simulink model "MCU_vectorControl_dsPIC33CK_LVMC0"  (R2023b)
settings: Solver=FixedStepDiscrete  StartTime=0.0  StopTime=10.0  FixedStep=5e-5  RelTol=1e-3  EnableMultiTasking=on
undefined symbols (not defined in the file or in its folder): A0, A4, ADC, address, also, AN0, AN1, as, B0, B2, below, Bias1, Bias2, bit, bits, BOR, C12, C13, C14, C7, C8, cause, Code, Communicate, control, counter, Custom, D11, D12, D13, D14, D2, D5, D6, D7, D9, dead, default, deviced, diff, disasserted, DiscIntNeverNeededParam, ECIO, ensure, events, faster, HS3, I, I2C, I2C1, I2C2, I2C3, illegalInstruction, Interval, inverter, is, IsSigned1, IsSigned2, kHz, Lowest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
libraries: simulink x55, MCHP_Blockset x25
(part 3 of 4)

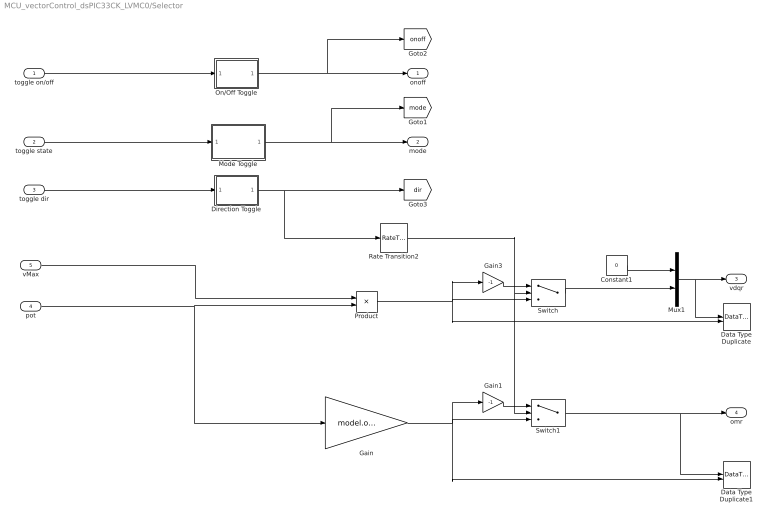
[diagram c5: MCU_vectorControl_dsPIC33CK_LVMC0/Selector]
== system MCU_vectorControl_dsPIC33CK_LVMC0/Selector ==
  toggle on/off : Inport  SampleTime=.01
  toggle state : Inport  Port=2  SampleTime=.01
  toggle dir : Inport  Port=3  SampleTime=.01
  pot : Inport  Port=4
  vMax : Inport  Port=5
  Constant1 : Constant  Value=0  OutDataTypeStr=Inherit: Inherit via back propagation
  Data Type Duplicate : DataTypeDuplicate
  Data Type Duplicate1 : DataTypeDuplicate
  Direction Toggle : Subsystem
  Gain : Gain  Gain=model.omegaMax  OutDataTypeStr=Inherit: Inherit via back propagation
  Gain1 : Gain  Gain=-1  OutDataTypeStr=Inherit: Inherit via back propagation  SaturateOnIntegerOverflow=on
  Gain3 : Gain  Gain=-1  OutDataTypeStr=Inherit: Inherit via back propagation  SaturateOnIntegerOverflow=on
  Mode Toggle : Subsystem
  Mux1 : Mux  Inputs=2
  On/Off Toggle : Subsystem
  Product : Product
  Rate Transition2 : RateTransition  Integrity=off  OutPortSampleTime=0.001
  Switch : Switch  Criteria=u2 > Threshold  OutDataTypeStr=Inherit: Inherit via back propagation
  Switch1 : Switch  Criteria=u2 > Threshold  OutDataTypeStr=Inherit: Inherit via back propagation
  onoff : Outport
  mode : Outport  Port=2
  vdqr : Outport  Port=3  VectorParamsAs1DForOutWhenUnconnected=off
  omr : Outport  Port=4  VectorParamsAs1DForOutWhenUnconnected=off
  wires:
  Switch1/1 -> omr/1, Data Type Duplicate1/1
  Direction Toggle/1(Toggle) -> Rate Transition2/1, [dir]
  Gain1/1 -> Switch1/1
  Gain/1 -> Gain1/1, Switch1/3, Data Type Duplicate1/2
  Product/1 -> Data Type Duplicate/2, Switch/3, Gain3/1
  Mux1/1 -> Data Type Duplicate/1, vdqr/1
  Constant1/1 -> Mux1/1
  toggle on/off/1 -> On/Off Toggle/1(in)
  On/Off Toggle/1(Toggle) -> [onoff], onoff/1
  Mode Toggle/1(Mode) -> [mode], mode/1
  toggle state/1 -> Mode Toggle/1(state)
  toggle dir/1 -> Direction Toggle/1(in)
  Gain3/1 -> Switch/1
  Switch/1 -> Mux1/2
  vMax/1 -> Product/1
  Rate Transition2/1 -> Switch/2, Switch1/2
  pot/1 -> Gain/1, Product/2

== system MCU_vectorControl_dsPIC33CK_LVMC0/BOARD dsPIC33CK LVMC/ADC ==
  ADC dsPIC High Speed SAR Motor Currents : MCHP_Blockset/Analog IO/ADC dsPIC High Speed SAR  ACLKCON=Optimized for PWM resolution & ADC conversion speed  ADC_FRACT=Fractional (left aligned)  ADC_NRE=off  DMA_Size=Single trigger - (default)  ADC_Synchronisation=Triggered by custom source  ADC_Trig_TXT=PWM1 Trigger 1  ADC_TrigTimeStep=Trig model step after all sample from this block are converted  ADC_TrigInfo=0  SampleTime=50e-6  S_INPUT=[]  S_INPUT_Size=[]  S_OUTPUT="[5  5]"  S_OUTPUT_Size="[1  1]"  S_ListCustomDatatype=S.S_ListCustomDatatype={};  MCHP_USER_INTERRUPTS={ADCAN0}{ADCBUF0}{ADC Data 0 Ready}{VectorName(ADCAN0Interrupt) Priority(-1) RegisterReadClear(ADCBUF0)Config_BitSet(ADIELbits.IE0) };{ADCAN1}{ADCBUF1}{ADC Data 1 Ready}{VectorName(ADCAN1Interrupt) Priority(-1) RegisterReadClear(ADCBUF1)Config_BitSet(ADIELbits.IE1) };  MCHP_PORT={Analog Input 0}{AN0}15:2:A0;{Analog Input 1}{AN1}15:2:B2;  MCHP_MASTERLINK=MCU_vectorControl_dsPIC33CK_LVMC0/BOARD dsPIC33CK LVMC/Microchip Master  MCHP_CRC=4309706  ADC_Info=Total Time = 640(ns)  ADC0_pin_TXT=AN0 / A0 / Pin[16]  ADC0_R="< 5    kOhm"  ADC0_res=12 bits  ADC0_signed=signed 16 bits  ADC0_FILTER=No Oversampling  ADC0_FILTER_nSamples=256 samples  ADC0_STRGEN=Start sampling followed by conversion  ADC0_STRGEN_on=Start sampling followed by conversion  ADC0_SSAMPEN=off  ADC0_Info=tSmp_min=260(ns) x 1 = 260(ns) ; tConv=370(ns) x 1 = 370(ns) ; TOTAL=640(ns)  ADC1_pin_TXT=AN1 / B2 / Pin[41]  ADC1_R="< 5    kOhm"  ADC1_res=12 bits  ADC1_signed=signed 16 bits  ADC1_FILTER=No Oversampling  ADC1_FILTER_nSamples=128 samples  ADC1_STRGEN=Start sampling followed by conversion  ADC1_STRGEN_on=Start sampling followed by conversion  ADC1_SSAMPEN=off  ADC1_Info=tSmp_min=260(ns) x 1 = 260(ns) ; tConv=370(ns) x 1 = 370(ns) ; TOTAL=640(ns)  ADC2_pin_TXT=Not used  ADC2_R="< 5    kOhm"  ADC2_res=12 bits  ADC2_signed=signed 16 bits  ADC2_FILTER=No Oversampling  ADC2_FILTER_nSamples=256 samples  ADC2_STRGEN=End sampling and start conversion  ADC2_STRGEN_on=Start sampling followed by conversion  ADC2_SSAMPEN=on  ADC2_Info=tSmp_min=14.706(ns) x 0 = 0(s) ; tConv=154.41(ns) x 0 = 0(s) ; TOTAL=0(s)  ADC3_pin_TXT=Not used  ADC3_R="< 10   kOhm"  ADC3_res=12 bits  ADC3_signed=signed 16 bits  ADC3_FILTER=Burst convert of n samples are Summed  ADC3_FILTER_nSamples=64 samples  ADC3_STRGEN=End sampling and start conversion  ADC3_STRGEN_on=Start sampling followed by conversion  ADC3_SSAMPEN=on  ADC3_Info=tSmp_min=14.706(ns) x 0 = 0(s) ; tConv=154.41(ns) x 0 = 0(s) ; TOTAL=0(s)  ADC4_pin_TXT=Not used  ADC4_R=< 200 Ohm  ADC4_res=12 bits  ADC4_signed=unsigned 16 bits  ADC4_FILTER=No Oversampling  ADC4_FILTER_nSamples=256 samples  ADC4_STRGEN=End sampling and start conversion  ADC4_STRGEN_on=Start sampling followed by conversion  ADC4_SSAMPEN=off  ADC4_Info=tSmp_min=14.706(ns) x 0 = 0(s) ; tConv=154.41(ns) x 0 = 0(s) ; TOTAL=0(s)  ADC5_pin_TXT=Not used  ADC5_R=< 200 Ohm  ADC5_res=12 bits  ADC5_signed=unsigned 16 bits  ADC5_FILTER=Burst convert of n samples are Summed  ADC5_FILTER_nSamples=256 samples  ADC5_STRGEN=End sampling and start conversion  ADC5_STRGEN_on=Start sampling followed by conversion  ADC5_SSAMPEN=on  ADC5_Info=tSmp_min=14.706(ns) x 0 = 0(s) ; tConv=154.41(ns) x 0 = 0(s) ; TOTAL=0(s)  ADC6_pin_TXT=Not used  ADC6_R=< 200 Ohm  ADC6_res=12 bits  ADC6_signed=unsigned 16 bits  ADC6_FILTER=Burst convert of n samples are Summed  ADC6_FILTER_nSamples=256 samples  ADC6_STRGEN=End sampling and start conversion  ADC6_STRGEN_on=Start sampling followed by conversion  ADC6_SSAMPEN=on  ADC6_Info=tSmp_min=14.706(ns) x 0 = 0(s) ; tConv=154.41(ns) x 0 = 0(s) ; TOTAL=0(s)  ADC7_R="< 5    kOhm"  ADC7_res=12 bits  ADC7_AN0=Not used  ADC7_AN1=Not used  ADC7_AN2=Not used  ADC7_AN3=Not used  ADC7_AN4=Not used  ADC7_AN5=Not used  ADC7_AN6=Not used  ADC7_AN7=Not used  ADC7_AN8=Not used  ADC7_AN9=Not used  ADC7_AN10=Not used  ADC7_AN11=Not used  ADC7_AN12=Not used  ADC7_AN13=Not used  ADC7_AN14=Not used  ADC7_AN15=Not used  ADC7_AN16=Not used  ADC7_AN17=Not used  ADC7_AN18=Not used  ADC7_AN19=Not used  ADC7_AN20=Not used  ADC7_AN21=Not used  ADC7_AN22=Not used  ADC7_AN23=Not used  ADC7_AN24=Not used  ADC7_AN25=Not used  ADC7_AN26=Not used  ADC7_AN27=Not used  ADC7_AN28=Not used  ADC7_AN29=Not used  ADC7_AN30=Not used  ADC7_AN31=Not used  IVref=Not used  IVTemp=Not used  ADC7_Info=tSmp_min=20(ns) x 0 = 0(s) ; tConv=210(ns) x 0 = 0(s) ; TOTAL=0(s)
  ADC dsPIC High Speed SAR others : MCHP_Blockset/Analog IO/ADC dsPIC High Speed SAR  ACLKCON=Not used  ADC_FRACT=Fractional (left aligned)  ADC_NRE=off  DMA_Size=Single trigger - (default)  ADC_Synchronisation=Triggered by custom source  ADC_Trig_TXT=PWM1 Trigger 1  ADC_TrigTimeStep=None (independant)  ADC_TrigInfo=0  SampleTime=50e-6  S_INPUT=[]  S_INPUT_Size=[]  S_OUTPUT="[5  5]"  S_OUTPUT_Size="[1  1]"  S_ListCustomDatatype=S.S_ListCustomDatatype={};  MCHP_USER_INTERRUPTS={ADCAN3}{ADCBUF3}{ADC Data 3 Ready}{VectorName(ADCAN3Interrupt) Priority(-1) RegisterReadClear(ADCBUF3)Config_BitSet(ADIELbits.IE3) };{ADCAN10}{ADCBUF10}{ADC Data 10 Ready}{VectorName(ADCAN10Interrupt) Priority(-1) RegisterReadClear(ADCBUF10)Config_BitSet(ADIELbits.IE10) };{ADCAN14}{ADCBUF14}{ADC Data 14 Ready}{VectorName(ADCAN14Interrupt) Priority(-1) RegisterReadClear(ADCBUF14)Config_BitSet(ADIE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  MCHP_PORT={Analog Input 4}{AN4}15:2:A4;{Analog Input 11}{AN11}15:2:B9;{Analog Input 15}{AN15}15:2:C3;  MCHP_MASTERLINK=MCU_vectorControl_dsPIC33CK_LVMC0/BOARD dsPIC33CK LVMC/Microchip Master  MCHP_CRC=4455074  ADC_Info=Total Time = 1.98(us)  ADC0_pin_TXT=Not used  ADC0_R="< 5    kOhm"  ADC0_res=12 bits  ADC0_signed=signed 16 bits  ADC0_FILTER=No Oversampling  ADC0_FILTER_nSamples=256 samples  ADC0_STRGEN=Start sampling followed by conversion  ADC0_STRGEN_on=Start sampling followed by conversion  ADC0_SSAMPEN=off  ADC0_Info=tSmp_min=20(ns) x 0 = 0(s) ; tConv=210(ns) x 0 = 0(s) ; TOTAL=0(s)  ADC1_pin_TXT=Not used  ADC1_R="< 5    kOhm"  ADC1_res=12 bits  ADC1_signed=signed 16 bits  ADC1_FILTER=No Oversampling  ADC1_FILTER_nSamples=128 samples  ADC1_STRGEN=Start sampling followed by conversion  ADC1_STRGEN_on=Start sampling followed by conversion  ADC1_SSAMPEN=off  ADC1_Info=tSmp_min=20(ns) x 0 = 0(s) ; tConv=210(ns) x 0 = 0(s) ; TOTAL=0(s)  ADC2_pin_TXT=Not used  ADC2_R="< 5    kOhm"  ADC2_res=12 bits  ADC2_signed=signed 16 bits  ADC2_FILTER=No Oversampling  ADC2_FILTER_nSamples=256 samples  ADC2_STRGEN=End sampling and start conversion  ADC2_STRGEN_on=Start sampling followed by conversion  ADC2_SSAMPEN=on  ADC2_Info=tSmp_min=14.706(ns) x 0 = 0(s) ; tConv=154.41(ns) x 0 = 0(s) ; TOTAL=0(s)  ADC3_pin_TXT=Not used  ADC3_R="< 10   kOhm"  ADC3_res=12 bits  ADC3_signed=signed 16 bits  ADC3_FILTER=Burst convert of n samples are Summed  ADC3_FILTER_nSamples=64 samples  ADC3_STRGEN=End sampling and start conversion  ADC3_STRGEN_on=Start sampling followed by conversion  ADC3_SSAMPEN=on  ADC3_Info=tSmp_min=14.706(ns) x 0 = 0(s) ; tConv=154.41(ns) x 0 = 0(s) ; TOTAL=0(s)  ADC4_pin_TXT=Not used  ADC4_R=< 200 Ohm  ADC4_res=12 bits  ADC4_signed=unsigned 16 bits  ADC4_FILTER=No Oversampling  ADC4_FILTER_nSamples=256 samples  ADC4_STRGEN=End sampling and start conversion  ADC4_STRGEN_on=Start sampling followed by conversion  ADC4_SSAMPEN=off  ADC4_Info=tSmp_min=14.706(ns) x 0 = 0(s) ; tConv=154.41(ns) x 0 = 0(s) ; TOTAL=0(s)  ADC5_pin_TXT=Not used  ADC5_R=< 200 Ohm  ADC5_res=12 bits  ADC5_signed=unsigned 16 bits  ADC5_FILTER=Burst convert of n samples are Summed  ADC5_FILTER_nSamples=256 samples  ADC5_STRGEN=End sampling and start conversion  ADC5_STRGEN_on=Start sampling followed by conversion  ADC5_SSAMPEN=on  ADC5_Info=tSmp_min=14.706(ns) x 0 = 0(s) ; tConv=154.41(ns) x 0 = 0(s) ; TOTAL=0(s)  ADC6_pin_TXT=Not used  ADC6_R=< 200 Ohm  ADC6_res=12 bits  ADC6_signed=unsigned 16 bits  ADC6_FILTER=Burst convert of n samples are Summed  ADC6_FILTER_nSamples=256 samples  ADC6_STRGEN=End sampling and start conversion  ADC6_STRGEN_on=Start sampling followed by conversion  ADC6_SSAMPEN=on  ADC6_Info=tSmp_min=14.706(ns) x 0 = 0(s) ; tConv=154.41(ns) x 0 = 0(s) ; TOTAL=0(s)  ADC7_R="< 5    kOhm"  ADC7_res=12 bits  ADC7_AN0=Not used  ADC7_AN1=Not used  ADC7_AN2=Not used  ADC7_AN3=Not used  ADC7_AN4=signed int16  ADC7_AN5=Not used  ADC7_AN6=Not used  ADC7_AN7=Not used  ADC7_AN8=Not used  ADC7_AN9=Not used  ADC7_AN10=Not used  ADC7_AN11=unsigned int16  ADC7_AN12=Not used  ADC7_AN13=Not used  ADC7_AN14=Not used  ADC7_AN15=unsigned int16  ADC7_AN16=Not used  ADC7_AN17=Not used  ADC7_AN18=Not used  ADC7_AN19=Not used  ADC7_AN20=Not used  ADC7_AN21=Not used  ADC7_AN22=Not used  ADC7_AN23=Not used  ADC7_AN24=Not used  ADC7_AN25=Not used  ADC7_AN26=Not used  ADC7_AN27=Not used  ADC7_AN28=Not used  ADC7_AN29=Not used  ADC7_AN30=Not used  ADC7_AN31=Not used  IVref=Not used  IVTemp=Not used  ADC7_Info=tSmp_min=280(ns) x 3 = 840(ns) ; tConv=370(ns) x 3 = 1.11(us) ; TOTAL=1.98(us)
  Ia : Outport  VectorParamsAs1DForOutWhenUnconnected=off
  Ib : Outport  Port=2  VectorParamsAs1DForOutWhenUnconnected=off
  IBus : Outport  Port=3  VectorParamsAs1DForOutWhenUnconnected=off
  pot : Outport  Port=4  VectorParamsAs1DForOutWhenUnconnected=off
  V_BUS : Outport  Port=5  VectorParamsAs1DForOutWhenUnconnected=off
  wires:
  ADC dsPIC High Speed SAR Motor Currents/2 -> Ib/1
  ADC dsPIC High Speed SAR Motor Currents/1 -> Ia/1
  ADC dsPIC High Speed SAR others/1 -> IBus/1
  ADC dsPIC High Speed SAR others/2 -> pot/1
  ADC dsPIC High Speed SAR others/3 -> V_BUS/1

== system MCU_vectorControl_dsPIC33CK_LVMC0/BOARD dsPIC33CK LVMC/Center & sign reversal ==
  I_ab : Inport
  Bias Update : Inport  Port=2
  Average and Sign reverse : Sum  Inputs=+-  SaturateOnIntegerOverflow=on
  Downsample Averaged 2000 samples remove bias : Subsystem  mask{DownSample=2000}
      mask prompts: DownSample "DownSample Factor"
  Rate Transition1 : RateTransition  Deterministic=off
  Iab : Outport
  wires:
  I_ab/1 -> Average and Sign reverse/2, Downsample Averaged 2000 samples remove bias/1(In1)
  Bias Update/1 -> Downsample Averaged 2000 samples remove bias/Enable
  Downsample Averaged 2000 samples remove bias/1(Out1) -> Rate Transition1/1
  Rate Transition1/1 -> Average and Sign reverse/1
  Average and Sign reverse/1 -> Iab/1  "I_ab_raw"

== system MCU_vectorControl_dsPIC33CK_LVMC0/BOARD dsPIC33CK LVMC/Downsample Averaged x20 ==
  note: DownSample & Average by changing data scaling
  In1 : Inport
  Compare To Constant : simulink/Logic and Bit Operations/Compare To Constant  relop===  const=1  OutDataTypeStr=boolean
  Counter Limited : simulink/Sources/Counter Limited  uplimit=DownSample-1  tsamp=-1
  Data Type Duplicate : DataTypeDuplicate
  Data Type Propagation : simulink/Signal Attributes/Data Type Propagation  PropDataType=fixdt(1, 16)  IfRefDouble=double  IfRefSingle=single  IsSigned=IsSigned1 or IsSigned2  NumBitsBase=NumBits1+NumBits2  NumBitsMult=1  NumBitsAdd=0  NumBitsAllowFinal=1:128  PropScaling=2^-10  ValuesUsedBestPrec=[5 -7]  SlopeBase=Slope1  SlopeMult=1  SlopeAdd=0  BiasBase=Bias1  BiasMult=1  BiasAdd=0
  Data Type Propagation1 : simulink/Signal Attributes/Data Type Propagation  PropDataType=fixdt(1, 16)  IfRefDouble=double  IfRefSingle=single  IsSigned=IsSigned1 or IsSigned2  NumBitsBase=NumBits1+NumBits2  NumBitsMult=1  NumBitsAdd=0  NumBitsAllowFinal=1:128  PropScaling=2^-10  ValuesUsedBestPrec=[5 -7]  SlopeBase=PosRange1  SlopeMult=1  SlopeAdd=0  BiasBase=Bias1  BiasMult=1  BiasAdd=0
  Discrete-Time Integrator : DiscreteIntegrator  IntegratorMethod=Accumulation: Backward Euler  gainval=1  ExternalReset=sampled level  SampleTime=-1  OutDataTypeStr=Inherit: Inherit via back propagation  ICPrevOutput=DiscIntNeverNeededParam  ICPrevScaledInput=DiscIntNeverNeededParam
  Gain : Gain  Gain=1/DownSample  OutDataTypeStr=Inherit: Inherit via back propagation  RndMeth=Round
  Gain1 : Gain  Gain=1/DownSample  OutDataTypeStr=Inherit: Inherit via back propagation
  Rate Transition1 : RateTransition  OutPortSampleTimeOpt=Multiple of input port sample time  OutPortSampleTimeMultiple=DownSample  OutPortSampleTime=DownSample
  Rate Transition3 : RateTransition  OutPortSampleTimeOpt=Multiple of input port sample time  OutPortSampleTimeMultiple=DownSample  OutPortSampleTime=DownSample
  Terminator : Terminator
  Out1 : Outport  VectorParamsAs1DForOutWhenUnconnected=off
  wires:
  Gain1/1 -> Data Type Propagation1/3, Terminator/1
  Rate Transition1/1 -> Data Type Duplicate/1, Data Type Propagation1/1, Data Type Propagation1/2
  Gain/1 -> Out1/1, Data Type Duplicate/2
  Counter Limited/1 -> Compare To Constant/1
  Discrete-Time Integrator/1 -> Rate Transition3/1, Data Type Propagation/3
  Compare To Constant/1 -> Discrete-Time Integrator/2
  In1/1 -> Data Type Propagation/1, Data Type Propagation/2, Discrete-Time Integrator/1, Rate Transition1/1
  Rate Transition3/1 -> Gain/1, Gain1/1

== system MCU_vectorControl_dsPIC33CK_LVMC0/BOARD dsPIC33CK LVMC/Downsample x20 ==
  note: DownSample & Average by changing data scaling
  In1 : Inport
  Compare To Constant : simulink/Logic and Bit Operations/Compare To Constant  relop===  const=1  OutDataTypeStr=boolean
  Counter Limited : simulink/Sources/Counter Limited  uplimit=DownSample-1  tsamp=-1
  Data Type Duplicate : DataTypeDuplicate
  Data Type Propagation : simulink/Signal Attributes/Data Type Propagation  PropDataType=fixdt(1, 16)  IfRefDouble=double  IfRefSingle=single  IsSigned=IsSigned1 or IsSigned2  NumBitsBase=NumBits1+NumBits2  NumBitsMult=1  NumBitsAdd=0  NumBitsAllowFinal=1:128  PropScaling=2^-10  ValuesUsedBestPrec=[5 -7]  SlopeBase=Slope1  SlopeMult=1  SlopeAdd=0  BiasBase=Bias1  BiasMult=1  BiasAdd=0
  Data Type Propagation1 : simulink/Signal Attributes/Data Type Propagation  PropDataType=fixdt(1, 16)  IfRefDouble=double  IfRefSingle=single  IsSigned=IsSigned1 or IsSigned2  NumBitsBase=NumBits1+NumBits2  NumBitsMult=1  NumBitsAdd=0  NumBitsAllowFinal=1:128  PropScaling=2^-10  ValuesUsedBestPrec=[5 -7]  SlopeBase=PosRange1  SlopeMult=1  SlopeAdd=0  BiasBase=Bias1  BiasMult=1  BiasAdd=0
  Discrete-Time Integrator : DiscreteIntegrator  IntegratorMethod=Accumulation: Backward Euler  gainval=1  ExternalReset=sampled level  SampleTime=-1  OutDataTypeStr=Inherit: Inherit via back propagation  ICPrevOutput=DiscIntNeverNeededParam  ICPrevScaledInput=DiscIntNeverNeededParam
  Gain : Gain  Gain=1/DownSample  OutDataTypeStr=Inherit: Inherit via back propagation  RndMeth=Round
  Gain1 : Gain  Gain=1/DownSample  OutDataTypeStr=Inherit: Inherit via back propagation
  Rate Transition1 : RateTransition  OutPortSampleTimeOpt=Multiple of input port sample time  OutPortSampleTimeMultiple=DownSample  OutPortSampleTime=DownSample
  Rate Transition3 : RateTransition  OutPortSampleTimeOpt=Multiple of input port sample time  OutPortSampleTimeMultiple=DownSample  OutPortSampleTime=DownSample
  Terminator : Terminator
  Out1 : Outport  VectorParamsAs1DForOutWhenUnconnected=off
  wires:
  Rate Transition3/1 -> Gain1/1, Gain/1
  In1/1 -> Rate Transition1/1, Discrete-Time Integrator/1, Data Type Propagation/2, Data Type Propagation/1
  Compare To Constant/1 -> Discrete-Time Integrator/2
  Discrete-Time Integrator/1 -> Data Type Propagation/3, Rate Transition3/1
  Counter Limited/1 -> Compare To Constant/1
  Gain/1 -> Data Type Duplicate/2, Out1/1
  Rate Transition1/1 -> Data Type Propagation1/2, Data Type Propagation1/1, Data Type Duplicate/1
  Gain1/1 -> Terminator/1, Data Type Propagation1/3

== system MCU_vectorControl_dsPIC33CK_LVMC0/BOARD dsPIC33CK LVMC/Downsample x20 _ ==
  note: DownSample & Average by changing data scaling
  In1 : Inport
  Compare To Constant : simulink/Logic and Bit Operations/Compare To Constant  relop===  const=1  OutDataTypeStr=boolean
  Counter Limited : simulink/Sources/Counter Limited  uplimit=DownSample-1  tsamp=-1
  Data Type Duplicate : DataTypeDuplicate
  Data Type Propagation : simulink/Signal Attributes/Data Type Propagation  PropDataType=fixdt(1, 16)  IfRefDouble=double  IfRefSingle=single  IsSigned=IsSigned1 or IsSigned2  NumBitsBase=NumBits1+NumBits2  NumBitsMult=1  NumBitsAdd=0  NumBitsAllowFinal=1:128  PropScaling=2^-10  ValuesUsedBestPrec=[5 -7]  SlopeBase=Slope1  SlopeMult=1  SlopeAdd=0  BiasBase=Bias1  BiasMult=1  BiasAdd=0
  Data Type Propagation1 : simulink/Signal Attributes/Data Type Propagation  PropDataType=fixdt(1, 16)  IfRefDouble=double  IfRefSingle=single  IsSigned=IsSigned1 or IsSigned2  NumBitsBase=NumBits1+NumBits2  NumBitsMult=1  NumBitsAdd=0  NumBitsAllowFinal=1:128  PropScaling=2^-10  ValuesUsedBestPrec=[5 -7]  SlopeBase=PosRange1  SlopeMult=1  SlopeAdd=0  BiasBase=Bias1  BiasMult=1  BiasAdd=0
  Discrete-Time Integrator : DiscreteIntegrator  IntegratorMethod=Accumulation: Backward Euler  gainval=1  ExternalReset=sampled level  SampleTime=-1  OutDataTypeStr=Inherit: Inherit via back propagation  ICPrevOutput=DiscIntNeverNeededParam  ICPrevScaledInput=DiscIntNeverNeededParam
  Gain : Gain  Gain=1/DownSample  OutDataTypeStr=Inherit: Inherit via back propagation  RndMeth=Round
  Gain1 : Gain  Gain=1/DownSample  OutDataTypeStr=Inherit: Inherit via back propagation
  Rate Transition1 : RateTransition  OutPortSampleTimeOpt=Multiple of input port sample time  OutPortSampleTimeMultiple=DownSample  OutPortSampleTime=DownSample
  Rate Transition3 : RateTransition  OutPortSampleTimeOpt=Multiple of input port sample time  OutPortSampleTimeMultiple=DownSample  OutPortSampleTime=DownSample
  Terminator : Terminator
  Out1 : Outport  VectorParamsAs1DForOutWhenUnconnected=off
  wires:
  Gain1/1 -> Data Type Propagation1/3, Terminator/1
  Rate Transition1/1 -> Data Type Duplicate/1, Data Type Propagation1/1, Data Type Propagation1/2
  Gain/1 -> Out1/1, Data Type Duplicate/2
  Counter Limited/1 -> Compare To Constant/1
  Discrete-Time Integrator/1 -> Rate Transition3/1, Data Type Propagation/3
  Compare To Constant/1 -> Discrete-Time Integrator/2
  In1/1 -> Data Type Propagation/1, Data Type Propagation/2, Discrete-Time Integrator/1, Rate Transition1/1
  Rate Transition3/1 -> Gain/1, Gain1/1

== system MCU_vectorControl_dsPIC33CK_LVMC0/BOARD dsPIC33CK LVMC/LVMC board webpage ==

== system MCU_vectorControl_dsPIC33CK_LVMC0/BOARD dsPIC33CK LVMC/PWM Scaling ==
  vabc [0 1] : Inport
  Gain : Gain  Gain=PWM1max  OutDataTypeStr=uint16
  PWM : Outport  VectorParamsAs1DForOutWhenUnconnected=off
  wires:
  vabc [0 1]/1 -> Gain/1
  Gain/1 -> PWM/1

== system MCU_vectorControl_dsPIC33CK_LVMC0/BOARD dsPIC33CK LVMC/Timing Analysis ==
  note: CPU overload is 0 if no overload took place between two MCU Overload block execution. Otherwise, bits field output code for TID(s) responsible for at least one overload.
  Downsample Averaged2 : Subsystem  mask{InputSampleTime=.0005, DownSample=200}
      mask prompts: InputSampleTime "Input sample time"; DownSample "DownSample Factor"
  Gain : Gain  Gain=10e-9/.0005 * 100  OutMin=0  OutMax=100  OutDataTypeStr=fixdt(0,16)  RndMeth=Simplest  SaturateOnIntegerOverflow=on
  MCU Load : MCHP_Blockset/Profiling/MCU Load  MCULoadPin_TXT=None  MCULoadMeasure=on  TIMER_Resolution_TXT="Resol: 0.01(us)  -  Max: 0.655(ms)"  MCHP_TIMER_REQUEST={MCU_Load}{MCU_Load}21:5:0:0:[]:65536;  MCHP_TIMER_RESULT=[1 65535 ]  MCHP_MASTERLINK=MCU_vectorControl_dsPIC33CK_LVMC0/BOARD dsPIC33CK LVMC/Microchip Master  MCHP_COMPILED_INFO="CompiledSampleTime= [0.00050000000000000001041   0 ];CompiledInportDataTypes=[    ];CompiledInportDataWidth=[];"  Info="Timer 1:  Resol: 10(ns)  -  Max: 655.36(us)"  SampleTime=.0005
  MCU Overload : MCHP_Blockset/Profiling/MCU Overload  MCUOverloadBlockOutput=on  MCUOverLoadPin_TXT=None  MCHP_MASTERLINK=MCU_vectorControl_dsPIC33CK_LVMC0/BOARD dsPIC33CK LVMC/Microchip Master  SampleTime=-1
  Overload : Constant  Value=65535  OutDataTypeStr=Inherit: Inherit via back propagation
  Rate Transition : RateTransition  Deterministic=off  OutPortSampleTime=.0005*200
  Switch : Switch  Criteria=u2 ~= 0
  CPU Load : Outport  Unit=%  SampleTime=.0005*200
  CPU Overload : Outport  Port=2
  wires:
  Rate Transition/1 -> Switch/2
  MCU Overload/1 -> Rate Transition/1, CPU Overload/1
  MCU Load/1 -> Downsample Averaged2/1(In1)
  Downsample Averaged2/1(Out1) -> Switch/3
  Switch/1 -> Gain/1
  Overload/1 -> Switch/1
  Gain/1 -> CPU Load/1

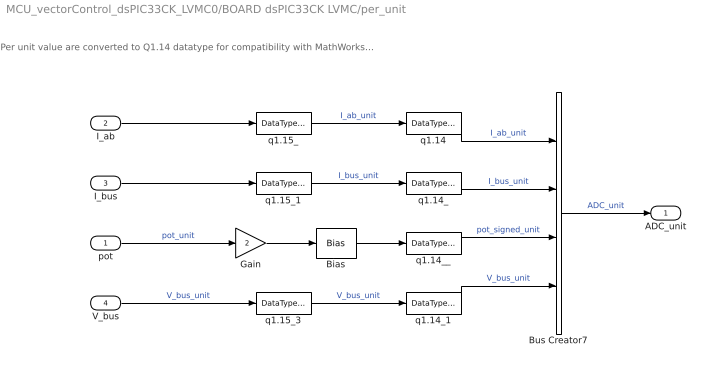
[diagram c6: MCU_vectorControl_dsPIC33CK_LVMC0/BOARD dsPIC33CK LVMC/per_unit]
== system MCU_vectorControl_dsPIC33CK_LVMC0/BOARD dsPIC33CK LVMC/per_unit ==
  note: Per unit value are converted to Q1.14 datatype for compatibility with MathWorks Motor Control Blockset (MCB)
  pot : Inport
  I_ab : Inport  Port=2
  I_bus : Inport  Port=3
  V_bus : Inport  Port=4
  Bias : Bias  Bias=-1
  Bus Creator7 : BusCreator  Inputs=4
  Gain : Gain  Gain=2  OutDataTypeStr=fixdt(1,16,15)
  q1.14 : DataTypeConversion  OutDataTypeStr=fixdt(1,16,14)
  q1.14_ : DataTypeConversion  OutDataTypeStr=fixdt(1,16,14)
  q1.14_1 : DataTypeConversion  OutDataTypeStr=fixdt(1,16,14)
  q1.14__ : DataTypeConversion  OutDataTypeStr=fixdt(1,16,14)
  q1.15_ : DataTypeConversion  OutDataTypeStr=fixdt(1,16,15)  ConvertRealWorld=Stored Integer (SI)
  q1.15_1 : DataTypeConversion  OutDataTypeStr=fixdt(1,16,15)  ConvertRealWorld=Stored Integer (SI)
  q1.15_3 : DataTypeConversion  OutDataTypeStr=fixdt(1,16,15)  ConvertRealWorld=Stored Integer (SI)
  ADC_unit : Outport
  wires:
  I_ab/1 -> q1.15_/1
  V_bus/1 -> q1.15_3/1  "V_bus_unit"
  pot/1 -> Gain/1  "pot_unit"
  I_bus/1 -> q1.15_1/1
  q1.15_1/1 -> q1.14_/1  "I_bus_unit"
  q1.15_/1 -> q1.14/1  "I_ab_unit"
  Bus Creator7/1 -> ADC_unit/1  "ADC_unit"
  q1.15_3/1 -> q1.14_1/1  "V_bus_unit"
  q1.14/1 -> Bus Creator7/1  "I_ab_unit"
  q1.14_/1 -> Bus Creator7/2  "I_bus_unit"
  q1.14__/1 -> Bus Creator7/3  "pot_signed_unit"
  q1.14_1/1 -> Bus Creator7/4  "V_bus_unit"
  Gain/1 -> Bias/1
  Bias/1 -> q1.14__/1

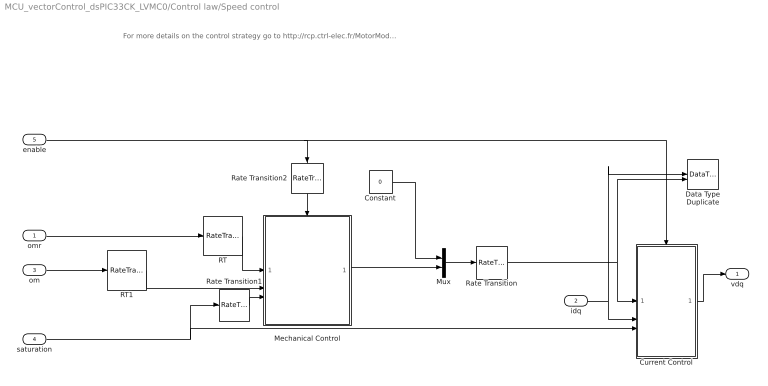
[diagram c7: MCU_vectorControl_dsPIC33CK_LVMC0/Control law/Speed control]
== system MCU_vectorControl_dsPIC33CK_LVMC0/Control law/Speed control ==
  note: For more details on the control strategy go to http://rcp.ctrl-elec.fr/MotorModeling/PMSMControl.html
  omr : Inport
  idq : Inport  Port=2
  om : Inport  Port=3
  saturation : Inport  Port=4
  enable : Inport  Port=5
  Constant : Constant  Value=0  OutDataTypeStr=Inherit: Inherit via back propagation
  Current Control : Subsystem
  Data Type Duplicate : DataTypeDuplicate
  Mechanical Control : Subsystem
  Mux : Mux  Inputs=2
  RT : RateTransition  OutPortSampleTime=0.001
  RT1 : RateTransition  OutPortSampleTime=0.001
  Rate Transition : RateTransition
  Rate Transition1 : RateTransition  OutPortSampleTime=control.tsMeca
  Rate Transition2 : RateTransition
  vdq : Outport
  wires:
  Rate Transition2/1 -> Mechanical Control/Enable
  enable/1 -> Rate Transition2/1, Current Control/Enable
  Rate Transition1/1 -> Mechanical Control/3(saturationV)
  omr/1 -> RT/1
  Rate Transition/1 -> Current Control/1(idqref), Data Type Duplicate/2
  Constant/1 -> Mux/1
  om/1 -> RT1/1
  saturation/1 -> Current Control/3(saturation), Rate Transition1/1
  Current Control/1(v) -> vdq/1
  Mux/1 -> Rate Transition/1
  idq/1 -> Current Control/2(idq), Data Type Duplicate/1
  RT/1 -> Mechanical Control/1(omref)
  RT1/1 -> Mechanical Control/2(om)
  Mechanical Control/1(iqref) -> Mux/2

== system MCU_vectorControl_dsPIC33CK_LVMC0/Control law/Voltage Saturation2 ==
  vdq : Inport
  vMax : Inport  Port=2
  1/sqrt(u) : Subsystem
  Data Type Duplicate : DataTypeDuplicate  NumInputPorts=3
  Divide : Product  Inputs=***  OutDataTypeStr=Inherit: Inherit via back propagation  SaturateOnIntegerOverflow=on
  Norm L2 : Subsystem
  Rate Transition : RateTransition
  Rate Transition1 : RateTransition
  Relational Operator : RelationalOperator  Operator=>  OutDataTypeStr=boolean  RndMeth=Simplest
  Square : Subsystem
  Sum : Sum  Inputs=|+-  OutDataTypeStr=Inherit: Inherit via back propagation  SaturateOnIntegerOverflow=on
  Switch : Switch  Criteria=u2 > Threshold  OutDataTypeStr=Inherit: Inherit via back propagation
  vdqsat : Outport  VectorParamsAs1DForOutWhenUnconnected=off
  saturation : Outport  Port=2  VectorParamsAs1DForOutWhenUnconnected=off
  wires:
  1/sqrt(u)/1(y) -> Divide/2
  Rate Transition1/1 -> Relational Operator/2
  Rate Transition/1 -> Divide/1
  Square/1(y) -> Rate Transition1/1
  vMax/1 -> Rate Transition/1, Square/1(In1)
  Relational Operator/1 -> Switch/2
  Sum/1 -> Data Type Duplicate/3, saturation/1
  vdq/1 -> Data Type Duplicate/1, Norm L2/1(In1), Divide/3, Switch/3, Sum/1
  Switch/1 -> Sum/2, Data Type Duplicate/2, vdqsat/1
  Norm L2/1(y) -> Relational Operator/1, 1/sqrt(u)/1(u)
  Divide/1 -> Switch/1

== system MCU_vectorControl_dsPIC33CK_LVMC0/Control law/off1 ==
  Mux : Mux  Inputs=2
  vd : Constant  Value=0  OutDataTypeStr=Inherit: Inherit via back propagation
  vq : Constant  Value=0  OutDataTypeStr=Inherit: Inherit via back propagation
  vdq : Outport  VectorParamsAs1DForOutWhenUnconnected=off
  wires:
  vq/1 -> Mux/2
  Mux/1 -> vdq/1
  vd/1 -> Mux/1

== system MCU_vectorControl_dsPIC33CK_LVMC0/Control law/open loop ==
  vdqr : Inport
  Enable : EnablePort
  vdq : Outport  VectorParamsAs1DForOutWhenUnconnected=off
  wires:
  vdqr/1 -> vdq/1

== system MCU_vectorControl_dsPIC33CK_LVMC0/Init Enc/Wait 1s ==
  Enable : EnablePort  StatesWhenEnabling=reset
  AND : Logic  IconShape=distinctive  AllPortsSameDT=off  OutDataTypeStr=boolean
  Compare To Constant : simulink/Logic and Bit Operations/Compare To Constant  relop=>  const=1  OutDataTypeStr=boolean
  Compare To Constant1 : simulink/Logic and Bit Operations/Compare To Constant  relop=>  const=1.1  OutDataTypeStr=boolean
  Constant1 : Constant  OutDataTypeStr=int16
  Discrete-Time Integrator : DiscreteIntegrator  SampleTime=-1  SaturateOnIntegerOverflow=on  LimitOutput=on  UpperSaturationLimit=2  LowerSaturationLimit=0  ICPrevOutput=DiscIntNeverNeededParam  ICPrevScaledInput=DiscIntNeverNeededParam
  NOT : Logic  Operator=NOT  IconShape=distinctive  AllPortsSameDT=off  OutDataTypeStr=boolean
  init enc : Outport
  init done : Outport  Port=2
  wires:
  NOT/1 -> AND/2
  AND/1 -> init enc/1
  Compare To Constant1/1 -> NOT/1, init done/1
  Discrete-Time Integrator/1 -> Compare To Constant/1, Compare To Constant1/1
  Constant1/1 -> Discrete-Time Integrator/1
  Compare To Constant/1 -> AND/1

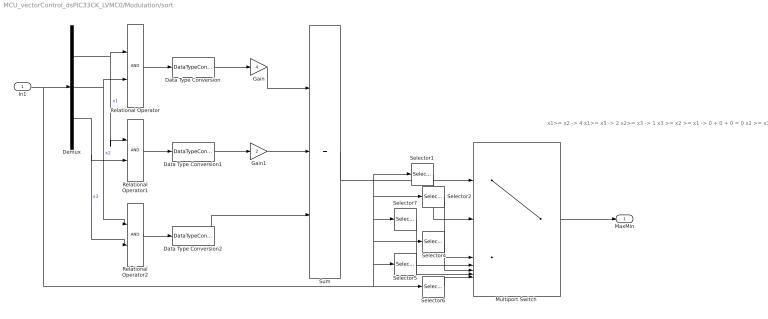
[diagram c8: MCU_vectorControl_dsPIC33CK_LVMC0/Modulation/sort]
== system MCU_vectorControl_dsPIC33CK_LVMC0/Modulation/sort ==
  note: x1>= x2 -> 4 x1>= x3 -> 2 x2>= x3 -> 1 x3 >= x2 >= x1 -> 0 + 0 + 0 = 0 x2 >= x3 >= x1 -> 0 + 0 + 1 = 1 x2 >= x1 >= x3 -> 0 + 2 + 1 = 3 x3 >= x1 >= x2 -> 4 + 0 + 0 = 4 x1 >= x3 >= x2 -> 4 + 2 + 0 = 6 x1 >= x2 >= x3 -> 4 + 2 + 1 = 7
  In1 : Inport
  Data Type Conversion : DataTypeConversion  OutDataTypeStr=int8
  Data Type Conversion1 : DataTypeConversion  OutDataTypeStr=int8
  Data Type Conversion2 : DataTypeConversion  OutDataTypeStr=int8
  Demux : Demux  Outputs=3
  Gain : Gain  Gain=4
  Gain1 : Gain  Gain=2
  Multiport Switch : MultiPortSwitch  DataPortOrder=Specify indices  DataPortIndices={0,1,3,4,6,7}
  Relational Operator : RelationalOperator  OutDataTypeStr=boolean  RndMeth=Simplest
  Relational Operator1 : RelationalOperator  OutDataTypeStr=boolean  RndMeth=Simplest
  Relational Operator2 : RelationalOperator  OutDataTypeStr=boolean  RndMeth=Simplest
  Selector1 : Selector  InputPortWidth=3  IndexOptions=Index vector (dialog)  Indices=[3 1]  OutputSizes=1
  Selector2 : Selector  InputPortWidth=3  IndexOptions=Index vector (dialog)  Indices=[2 1]  OutputSizes=1
  Selector4 : Selector  InputPortWidth=3  IndexOptions=Index vector (dialog)  Indices=[3 2]  OutputSizes=1
  Selector5 : Selector  InputPortWidth=3  IndexOptions=Index vector (dialog)  Indices=[1 2]  OutputSizes=1
  Selector6 : Selector  InputPortWidth=3  IndexOptions=Index vector (dialog)  Indices=[1 3]  OutputSizes=1
  Selector7 : Selector  InputPortWidth=3  IndexOptions=Index vector (dialog)  Indices=[2 3]  OutputSizes=1
  Sum : Sum  Inputs=+++
  MaxMin : Outport
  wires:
  Multiport Switch/1 -> MaxMin/1
  Selector2/1 -> Multiport Switch/3
  Selector7/1 -> Multiport Switch/4
  Selector4/1 -> Multiport Switch/5
  Selector5/1 -> Multiport Switch/6
  Selector6/1 -> Multiport Switch/7
  Selector1/1 -> Multiport Switch/2
  Sum/1 -> Multiport Switch/1
  Data Type Conversion2/1 -> Sum/3
  Gain/1 -> Sum/1
  Gain1/1 -> Sum/2
  Data Type Conversion1/1 -> Gain1/1
  Data Type Conversion/1 -> Gain/1
  Relational Operator/1 -> Data Type Conversion/1
  Relational Operator1/1 -> Data Type Conversion1/1
  Relational Operator2/1 -> Data Type Conversion2/1
  In1/1 -> Demux/1, Selector6/1, Selector5/1, Selector1/1, Selector2/1, Selector7/1, Selector4/1
  Demux/1 -> Relational Operator/1, Relational Operator1/1  "x1"
  Demux/2 -> Relational Operator/2, Relational Operator2/1  "x2"
  Demux/3 -> Relational Operator1/2, Relational Operator2/2  "x3"

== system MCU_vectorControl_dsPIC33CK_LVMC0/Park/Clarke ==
  note: Clark transform $x_{\alpha\beta} = \frac{2}{3}\underbrace{\left[\begin{array}{ccc}1&-\frac{1}{2}&-\frac{1}{2}\\0&\frac{\sqrt{3}}{2}&-\frac{\sqrt{3}}{2}\end{array}\right]}_{C_{23}}x_{abc}$ if only 2 currents are measured since $x_a+x_b+x_c = 0$ $x_{abc} = \left[\begin{array}{cc}1 & 0\\0 & 1\\-1&-1\end{array}\right]x_{ab}$ leading to $x_{\alpha\beta} = \underbrace{\left[\begin{array}{cc}1&0\\\frac{1}{\sqrt{3}}&\frac{2}{\sqrt{3}}\end{array}\right]}_{C_{22}}x_{ab}$
  xab(c) : Inport
  C1 : Gain  Gain=[1/sqrt(3) 2/sqrt(3)]  Multiplication=Matrix(K*u)
  Mux : Mux  Inputs=2
  Selector : Selector  InputPortWidth=2  IndexOptions=Index vector (dialog)  Indices=[1]  OutputSizes=1
  xalphabeta : Outport  VectorParamsAs1DForOutWhenUnconnected=off
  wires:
  C1/1 -> Mux/2
  Selector/1 -> Mux/1
  Mux/1 -> xalphabeta/1
  xab(c)/1 -> C1/1, Selector/1

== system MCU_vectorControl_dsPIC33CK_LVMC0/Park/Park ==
  note: Park $x_{dq} = P(\theta)^{-1}x_{\alpha\beta}\\ P(p\theta)^{-1} = \left[\begin{array}{cc}\cos(p\theta) & \sin(p\theta)\\ -\sin(p\theta) & \cos(p\theta) \end{array}\right]$
  xalphabeta : Inport  PortDimensions=2
  P(pth) : Inport  Port=2
  Data Type Duplicate2 : DataTypeDuplicate
  Park : Product  Multiplication=Matrix(*)  OutDataTypeStr=Inherit: Inherit via back propagation  RndMeth=Round
  xdq : Outport  VectorParamsAs1DForOutWhenUnconnected=off
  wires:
  P(pth)/1 -> Park/1
  xalphabeta/1 -> Park/2, Data Type Duplicate2/2
  Park/1 -> xdq/1, Data Type Duplicate2/1

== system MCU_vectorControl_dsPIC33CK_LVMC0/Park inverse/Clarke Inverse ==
  note: Clarke inverse
  xalphabeta : Inport
  C23' : Gain  Gain=|  Multiplication=Matrix(K*u)  OutDataTypeStr=Inherit: Inherit via back propagation  RndMeth=Round
      | [1   -1/2        -1/2;
      |         0   sqrt(3)/2   -sqrt(3)/2]'
  xabc : Outport  VectorParamsAs1DForOutWhenUnconnected=off
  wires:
  xalphabeta/1 -> C23'/1
  C23'/1 -> xabc/1

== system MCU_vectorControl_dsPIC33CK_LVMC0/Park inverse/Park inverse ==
  note: Inverse Park $x_{\alpha\beta} = P(p\theta)x_{dq}\\ P(p\theta) = \left[\begin{array}{cc}\cos(p\theta) & -\sin(p\theta)\\ \sin(p\theta) & \cos(p\theta) \end{array}\right]$
  xdq : Inport
  P(pth) : Inport  Port=2
  Data Type Duplicate2 : DataTypeDuplicate
  Transpose : Math  Operator=transpose
  Transpose1 : Math  Operator=transpose
  xalpha sin(pth)1 : Product  Multiplication=Matrix(*)  OutDataTypeStr=Inherit: Inherit via back propagation  RndMeth=Round
  xalpahbeta : Outport  VectorParamsAs1DForOutWhenUnconnected=off
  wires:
  P(pth)/1 -> xalpha sin(pth)1/2
  Transpose1/1 -> xalpahbeta/1
  Transpose/1 -> Data Type Duplicate2/2, xalpha sin(pth)1/1
  xdq/1 -> Transpose/1
  xalpha sin(pth)1/1 -> Data Type Duplicate2/1, Transpose1/1

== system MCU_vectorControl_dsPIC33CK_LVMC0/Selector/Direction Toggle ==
  in : Inport
  Change when button is pressed : simulink/Logic and Bit Operations/Detect Decrease  vinit=0.0  OutDataTypeStr=uint8
  Logical Operator : Logic  Operator=XOR  AllPortsSameDT=off  OutDataTypeStr=boolean
  Unit Delay : UnitDelay  SampleTime=-1  HasFrameUpgradeWarning=on
  Toggle : Outport  VectorParamsAs1DForOutWhenUnconnected=off
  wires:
  Logical Operator/1 -> Unit Delay/1, Toggle/1  "Toggle"
  in/1 -> Change when button is pressed/1
  Change when button is pressed/1 -> Logical Operator/1
  Unit Delay/1 -> Logical Operator/2

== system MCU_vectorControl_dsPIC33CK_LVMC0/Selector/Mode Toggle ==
  state : Inport
  Bitwise Operator : simulink/Logic and Bit Operations/Bitwise Operator  logicop=AND  UseBitMask=on  BitMask=1  BitMaskRealWorld=Stored Integer
  Change when button is pressed : simulink/Logic and Bit Operations/Detect Decrease  vinit=0.0  OutDataTypeStr=uint8
  Sum : Sum  OutDataTypeStr=uint16  AccumDataTypeStr=uint16
  Unit Delay : UnitDelay  SampleTime=-1  HasFrameUpgradeWarning=on
  Mode : Outport  PortDimensions=1  VectorParamsAs1DForOutWhenUnconnected=off
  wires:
  Change when button is pressed/1 -> Sum/1
  Bitwise Operator/1 -> Mode/1, Unit Delay/1
  Unit Delay/1 -> Sum/2
  Sum/1 -> Bitwise Operator/1
  state/1 -> Change when button is pressed/1

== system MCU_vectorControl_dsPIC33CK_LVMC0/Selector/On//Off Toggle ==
  in : Inport
  Change when button is pressed : simulink/Logic and Bit Operations/Detect Decrease  vinit=0.0  OutDataTypeStr=uint8
  Logical Operator : Logic  Operator=XOR  AllPortsSameDT=off  OutDataTypeStr=boolean
  Unit Delay : UnitDelay  SampleTime=-1  HasFrameUpgradeWarning=on
  Toggle : Outport  VectorParamsAs1DForOutWhenUnconnected=off
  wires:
  Unit Delay/1 -> Logical Operator/2
  Change when button is pressed/1 -> Logical Operator/1
  in/1 -> Change when button is pressed/1
  Logical Operator/1 -> Unit Delay/1, Toggle/1  "Toggle"

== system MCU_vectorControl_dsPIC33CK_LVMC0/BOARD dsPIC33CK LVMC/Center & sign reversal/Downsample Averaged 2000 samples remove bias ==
  note: DownSample & Average by changing data scaling
  In1 : Inport
  Enable : EnablePort
  Compare To Constant : simulink/Logic and Bit Operations/Compare To Constant  relop===  const=1  OutDataTypeStr=boolean
  Counter Limited : simulink/Sources/Counter Limited  uplimit=DownSample-1  tsamp=-1
  Data Type Duplicate : DataTypeDuplicate
  Data Type Propagation : simulink/Signal Attributes/Data Type Propagation  PropDataType=fixdt(1, 16)  IfRefDouble=double  IfRefSingle=single  IsSigned=IsSigned1 or IsSigned2  NumBitsBase=NumBits1+NumBits2  NumBitsMult=1  NumBitsAdd=0  NumBitsAllowFinal=1:128  PropScaling=2^-10  ValuesUsedBestPrec=[5 -7]  SlopeBase=Slope1  SlopeMult=1  SlopeAdd=0  BiasBase=Bias1  BiasMult=1  BiasAdd=0
  Data Type Propagation1 : simulink/Signal Attributes/Data Type Propagation  PropDataType=fixdt(1, 16)  IfRefDouble=double  IfRefSingle=single  IsSigned=IsSigned1 or IsSigned2  NumBitsBase=NumBits1+NumBits2  NumBitsMult=1  NumBitsAdd=0  NumBitsAllowFinal=1:128  PropScaling=2^-10  ValuesUsedBestPrec=[5 -7]  SlopeBase=PosRange1  SlopeMult=1  SlopeAdd=0  BiasBase=Bias1  BiasMult=1  BiasAdd=0
  Discrete-Time Integrator : DiscreteIntegrator  IntegratorMethod=Accumulation: Backward Euler  gainval=1  ExternalReset=sampled level  SampleTime=-1  OutDataTypeStr=Inherit: Inherit via back propagation  ICPrevOutput=DiscIntNeverNeededParam  ICPrevScaledInput=DiscIntNeverNeededParam
  Gain : Gain  Gain=1/DownSample  OutDataTypeStr=Inherit: Inherit via back propagation  RndMeth=Round
  Gain1 : Gain  Gain=1/DownSample  OutDataTypeStr=Inherit: Inherit via back propagation
  Rate Transition1 : RateTransition  OutPortSampleTimeOpt=Multiple of input port sample time  OutPortSampleTimeMultiple=DownSample  OutPortSampleTime=DownSample
  Rate Transition3 : RateTransition  OutPortSampleTimeOpt=Multiple of input port sample time  OutPortSampleTimeMultiple=DownSample  OutPortSampleTime=DownSample
  Terminator : Terminator
  Out1 : Outport  VectorParamsAs1DForOutWhenUnconnected=off
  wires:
  Gain1/1 -> Data Type Propagation1/3, Terminator/1
  Rate Transition1/1 -> Data Type Duplicate/1, Data Type Propagation1/1, Data Type Propagation1/2
  Gain/1 -> Out1/1, Data Type Duplicate/2
  Counter Limited/1 -> Compare To Constant/1
  Discrete-Time Integrator/1 -> Rate Transition3/1, Data Type Propagation/3
  Compare To Constant/1 -> Discrete-Time Integrator/2
  In1/1 -> Data Type Propagation/1, Data Type Propagation/2, Discrete-Time Integrator/1, Rate Transition1/1
  Rate Transition3/1 -> Gain/1, Gain1/1

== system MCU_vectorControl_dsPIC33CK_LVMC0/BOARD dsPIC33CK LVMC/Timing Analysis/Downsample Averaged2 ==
  note: DownSample & Average by changing data scaling
  In1 : Inport
  Compare To Constant : simulink/Logic and Bit Operations/Compare To Constant  relop===  const=1  OutDataTypeStr=boolean
  Counter Limited : simulink/Sources/Counter Limited  uplimit=DownSample-1  tsamp=-1
  Data Type Duplicate : DataTypeDuplicate
  Data Type Propagation : simulink/Signal Attributes/Data Type Propagation  PropDataType=fixdt(1, 16)  IfRefDouble=double  IfRefSingle=single  IsSigned=IsSigned1 or IsSigned2  NumBitsBase=NumBits1+NumBits2  NumBitsMult=1  NumBitsAdd=0  NumBitsAllowFinal=1:128  PropScaling=2^-10  ValuesUsedBestPrec=[5 -7]  SlopeBase=Slope1  SlopeMult=1  SlopeAdd=0  BiasBase=Bias1  BiasMult=1  BiasAdd=0
  Data Type Propagation1 : simulink/Signal Attributes/Data Type Propagation  PropDataType=fixdt(1, 16)  IfRefDouble=double  IfRefSingle=single  IsSigned=IsSigned1 or IsSigned2  NumBitsBase=NumBits1+NumBits2  NumBitsMult=1  NumBitsAdd=0  NumBitsAllowFinal=1:128  PropScaling=2^-10  ValuesUsedBestPrec=[5 -7]  SlopeBase=PosRange1  SlopeMult=1  SlopeAdd=0  BiasBase=Bias1  BiasMult=1  BiasAdd=0
  Discrete-Time Integrator : DiscreteIntegrator  IntegratorMethod=Accumulation: Backward Euler  gainval=1  ExternalReset=sampled level  SampleTime=-1  OutDataTypeStr=Inherit: Inherit via back propagation  ICPrevOutput=DiscIntNeverNeededParam  ICPrevScaledInput=DiscIntNeverNeededParam
  Gain : Gain  Gain=1/DownSample  OutDataTypeStr=Inherit: Inherit via back propagation
  Gain1 : Gain  Gain=1/DownSample  OutDataTypeStr=Inherit: Inherit via back propagation
  Rate Transition1 : RateTransition  Deterministic=off  OutPortSampleTime=[InputSampleTime * DownSample]
  Rate Transition3 : RateTransition  OutPortSampleTime=[InputSampleTime * DownSample]
  Terminator : Terminator
  Out1 : Outport  VectorParamsAs1DForOutWhenUnconnected=off
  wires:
  Rate Transition3/1 -> Gain1/1, Gain/1
  In1/1 -> Discrete-Time Integrator/1, Rate Transition1/1, Data Type Propagation/2, Data Type Propagation/1
  Compare To Constant/1 -> Discrete-Time Integrator/2
  Discrete-Time Integrator/1 -> Data Type Propagation/3, Rate Transition3/1
  Counter Limited/1 -> Compare To Constant/1
  Gain/1 -> Data Type Duplicate/2, Out1/1
  Rate Transition1/1 -> Data Type Propagation1/2, Data Type Propagation1/1, Data Type Duplicate/1
  Gain1/1 -> Data Type Propagation1/3, Terminator/1

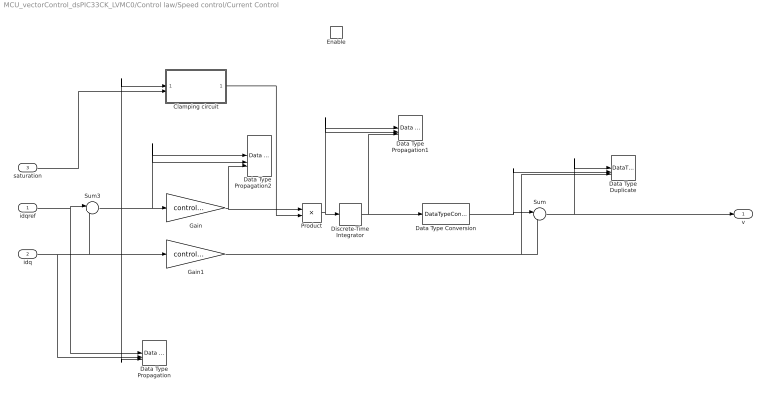
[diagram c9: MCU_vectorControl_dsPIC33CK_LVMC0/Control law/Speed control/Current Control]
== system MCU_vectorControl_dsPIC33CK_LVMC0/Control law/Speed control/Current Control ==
  idqref : Inport
  idq : Inport  Port=2
  saturation : Inport  Port=3
  Enable : EnablePort  StatesWhenEnabling=reset
  Clamping circuit : Subsystem
  Data Type Duplicate : DataTypeDuplicate  NumInputPorts=3
  Data Type Propagation : simulink/Signal Attributes/Data Type Propagation  PropDataType=fixdt(1, 16)  IfRefDouble=double  IfRefSingle=single  IsSigned=IsSigned1 or IsSigned2  NumBitsBase=max([NumBits1 NumBits2])  NumBitsMult=1  NumBitsAdd=0  NumBitsAllowFinal=1:128  PropScaling=2^-(15-ceil(log2(2*inverter.iMax)))  ValuesUsedBestPrec=[5 -7]  SlopeBase=max([PosRange1 PosRange2])  SlopeMult=2  SlopeAdd=0  BiasBase=Bias1  BiasMult=1  BiasAdd=0
  Data Type Propagation1 : simulink/Signal Attributes/Data Type Propagation  PropDataType=fixdt(1, 16)  IfRefDouble=single  IfRefSingle=single  IsSigned=IsSigned1 or IsSigned2  NumBitsBase=NumBits1+NumBits2  NumBitsMult=1  NumBitsAdd=0  NumBitsAllowFinal=1:128  PropScalingMode=Specify via dialog  PropScaling=2^-23  ValuesUsedBestPrec=[5 -7]  SlopeBase=min([Slope1 Slope2])  SlopeMult=1  SlopeAdd=0  BiasBase=Bias1  BiasMult=1  BiasAdd=0
  Data Type Propagation2 : simulink/Signal Attributes/Data Type Propagation  PropDataType=fixdt(1, 16)  IfRefDouble=double  IfRefSingle=single  IsSigned=TRUE  NumBitsBase=max([NumBits1 NumBits2])  NumBitsMult=1  NumBitsAdd=0  NumBitsAllowFinal=[1:128]  PropScaling=2^-(15-ceil(log2(inverter.vDC/sqrt(3))))  ValuesUsedBestPrec=[100 -100]  SlopeBase=max([PosRange1 PosRange2])  SlopeMult=abs(control.kE(2))  SlopeAdd=0  BiasBase=Bias1  BiasMult=1  BiasAdd=0
  Data Type Conversion : DataTypeConversion
  Discrete-Time Integrator : DiscreteIntegrator  SampleTime=-1  OutDataTypeStr=Inherit: Inherit via back propagation  SaturateOnIntegerOverflow=on  ICPrevOutput=DiscIntNeverNeededParam  ICPrevScaledInput=DiscIntNeverNeededParam
  Gain : Gain  Gain=control.kE(2)  OutDataTypeStr=Inherit: Inherit via back propagation  SaturateOnIntegerOverflow=on
  Gain1 : Gain  Gain=control.kE(1)  OutDataTypeStr=Inherit: Inherit via back propagation  SaturateOnIntegerOverflow=on
  Product : Product
  Sum : Sum  Inputs=|--  OutDataTypeStr=Inherit: Inherit via back propagation  SaturateOnIntegerOverflow=on
  Sum3 : Sum  Inputs=|+-  OutDataTypeStr=Inherit: Inherit via back propagation  SaturateOnIntegerOverflow=on
  v : Outport  VectorParamsAs1DForOutWhenUnconnected=off
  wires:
  Data Type Conversion/1 -> Sum/1, Data Type Duplicate/2
  Sum/1 -> v/1, Data Type Duplicate/1
  idqref/1 -> Sum3/1, Data Type Propagation/1
  idq/1 -> Sum3/2, Gain1/1, Data Type Propagation/2
  Discrete-Time Integrator/1 -> Data Type Conversion/1, Data Type Propagation1/3
  Gain1/1 -> Sum/2, Data Type Duplicate/3
  saturation/1 -> Clamping circuit/2(saturation)
  Product/1 -> Data Type Propagation1/2, Data Type Propagation1/1, Discrete-Time Integrator/1
  Clamping circuit/1(Clamp) -> Product/2
  Gain/1 -> Data Type Propagation2/3, Product/1
  Sum3/1 -> Gain/1, Data Type Propagation2/2, Data Type Propagation2/1, Data Type Propagation/3, Clamping circuit/1(preIntegrator)

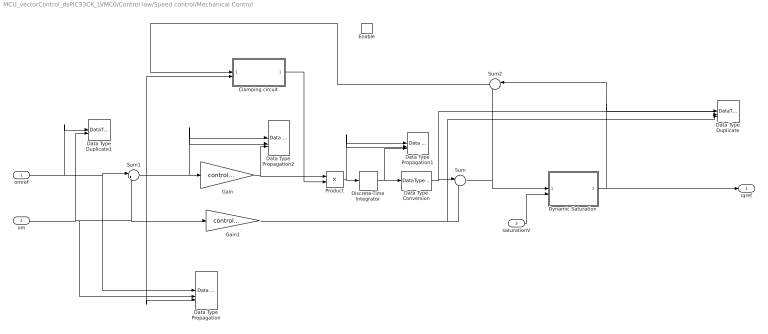
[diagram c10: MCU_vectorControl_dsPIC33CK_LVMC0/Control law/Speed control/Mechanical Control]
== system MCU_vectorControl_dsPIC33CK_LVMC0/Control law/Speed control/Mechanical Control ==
  omref : Inport
  om : Inport  Port=2
  saturationV : Inport  Port=3
  Enable : EnablePort  StatesWhenEnabling=reset
  Clamping circuit : Subsystem
  Data Type Duplicate : DataTypeDuplicate  NumInputPorts=3
  Data Type Duplicate1 : DataTypeDuplicate
  Data Type Propagation : simulink/Signal Attributes/Data Type Propagation  PropDataType=fixdt(1, 16)  IfRefDouble=double  IfRefSingle=single  IsSigned=IsSigned1 or IsSigned2  NumBitsBase=max([NumBits1 NumBits2])  NumBitsMult=1  NumBitsAdd=0  NumBitsAllowFinal=1:128  PropScaling=2^-(15-ceil(log2(2*pmsm.omegaMax)))  ValuesUsedBestPrec=[5 -7]  SlopeBase=max([PosRange1 PosRange2])  SlopeMult=2  SlopeAdd=0  BiasBase=Bias1  BiasMult=1  BiasAdd=0
  Data Type Propagation1 : simulink/Signal Attributes/Data Type Propagation  PropDataType=fixdt(1, 16)  IfRefDouble=single  IfRefSingle=single  IsSigned=IsSigned1 or IsSigned2  NumBitsBase=NumBits1+NumBits2  NumBitsMult=1  NumBitsAdd=0  NumBitsAllowFinal=1:128  PropScalingMode=Specify via dialog  PropScaling=2^-23  ValuesUsedBestPrec=[5 -7]  SlopeBase=min([Slope1 Slope2])  SlopeMult=1  SlopeAdd=0  BiasBase=Bias1  BiasMult=1  BiasAdd=0
  Data Type Propagation2 : simulink/Signal Attributes/Data Type Propagation  PropDataType=fixdt(1, 16)  IfRefDouble=double  IfRefSingle=single  IsSigned=TRUE  NumBitsBase=max([NumBits1 NumBits2])  NumBitsMult=1  NumBitsAdd=0  NumBitsAllowFinal=[1:128]  PropScaling=2^-(15-ceil(log2(inverter.vDC/sqrt(3))))  ValuesUsedBestPrec=[100 -100]  SlopeBase=max([PosRange1 PosRange2])  SlopeMult=abs(control.kM(2))  SlopeAdd=0  BiasBase=Bias1  BiasMult=1  BiasAdd=0
  Data Type Conversion : DataTypeConversion
  Discrete-Time Integrator : DiscreteIntegrator  SampleTime=-1  OutDataTypeStr=Inherit: Inherit via back propagation  SaturateOnIntegerOverflow=on  ICPrevOutput=DiscIntNeverNeededParam  ICPrevScaledInput=DiscIntNeverNeededParam
  Dynamic Saturation : Subsystem
  Gain : Gain  Gain=control.kM(2)  OutDataTypeStr=Inherit: Inherit via back propagation  SaturateOnIntegerOverflow=on
  Gain1 : Gain  Gain=control.kM(1)  OutDataTypeStr=Inherit: Inherit via back propagation  SaturateOnIntegerOverflow=on
  Product : Product
  Sum : Sum  Inputs=|--  OutDataTypeStr=Inherit: Inherit via back propagation  SaturateOnIntegerOverflow=on
  Sum1 : Sum  Inputs=|+-  OutDataTypeStr=Inherit: Inherit via back propagation
  Sum2 : Sum  Inputs=|-+  SaturateOnIntegerOverflow=on
  iqref : Outport  VectorParamsAs1DForOutWhenUnconnected=off
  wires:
  Data Type Conversion/1 -> Sum/1, Data Type Duplicate/2
  Dynamic Saturation/1(y) -> Sum2/1, Data Type Duplicate/1, iqref/1
  Sum/1 -> Sum2/2, Dynamic Saturation/1(u)
  Discrete-Time Integrator/1 -> Data Type Conversion/1, Data Type Propagation1/3
  om/1 -> Data Type Duplicate1/2, Sum1/2, Gain1/1, Data Type Propagation/2
  omref/1 -> Sum1/1, Data Type Propagation/1, Data Type Duplicate1/1
  Clamping circuit/1(Clamp) -> Product/2
  Sum2/1 -> Clamping circuit/1(Saturation)
  Gain1/1 -> Sum/2, Data Type Duplicate/3
  saturationV/1 -> Dynamic Saturation/2(saturationV)
  Product/1 -> Data Type Propagation1/2, Data Type Propagation1/1, Discrete-Time Integrator/1
  Gain/1 -> Data Type Propagation2/3, Product/1
  Sum1/1 -> Data Type Propagation2/1, Data Type Propagation2/2, Gain/1, Clamping circuit/2(preIntegrator), Data Type Propagation/3

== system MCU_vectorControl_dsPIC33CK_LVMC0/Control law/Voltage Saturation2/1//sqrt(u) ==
  u : Inport
  Calc 1/sqrt(u) : Subsystem
  Compare To Constant : simulink/Logic and Bit Operations/Compare To Constant  relop===  const=1  OutDataTypeStr=boolean
  Compare To Constant1 : simulink/Logic and Bit Operations/Compare To Constant  relop===  const=0  OutDataTypeStr=boolean
  "LUT 1/sqrt(u) " : Subsystem
  Switch : Switch  Criteria=u2 > Threshold
  isSingle : Subsystem
  y : Outport
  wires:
  Compare To Constant/1 -> Calc 1/sqrt(u)/Enable
  Compare To Constant1/1 -> "LUT 1/sqrt(u) "/Enable
  Switch/1 -> y/1
  "LUT 1/sqrt(u) "/1(vdqsat1) -> Switch/3
  Calc 1/sqrt(u)/1(Out1) -> Switch/1
  isSingle/1(y) -> Switch/2, Compare To Constant/1, Compare To Constant1/1
  u/1 -> "LUT 1/sqrt(u) "/1(y), isSingle/1(u), Calc 1/sqrt(u)/1(u)

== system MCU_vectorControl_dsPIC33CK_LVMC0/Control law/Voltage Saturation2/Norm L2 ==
  In1 : Inport
  Data Type Propagation : simulink/Signal Attributes/Data Type Propagation  PropDataType=fixdt(1, 16)  IfRefDouble=double  IfRefSingle=single  IsSigned=IsSigned1 or IsSigned2  NumBitsBase=max([NumBits1 NumBits2])  NumBitsMult=1  NumBitsAdd=0  NumBitsAllowFinal=1:128  PropScalingMode=Specify via dialog  PropScaling=2^-model.FracLen.volt2  ValuesUsedBestPrec=[5 -7]  SlopeBase=PosRange1*PosRange2  SlopeMult=1  SlopeAdd=0  BiasBase=max([Bias1 Bias2])  BiasMult=1  BiasAdd=0
  Dot Product : DotProduct  OutDataTypeStr=Inherit: Inherit via back propagation  SaturateOnIntegerOverflow=on
  y : Outport
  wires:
  In1/1 -> Data Type Propagation/1, Data Type Propagation/2, Dot Product/2, Dot Product/1
  Dot Product/1 -> Data Type Propagation/3, y/1
